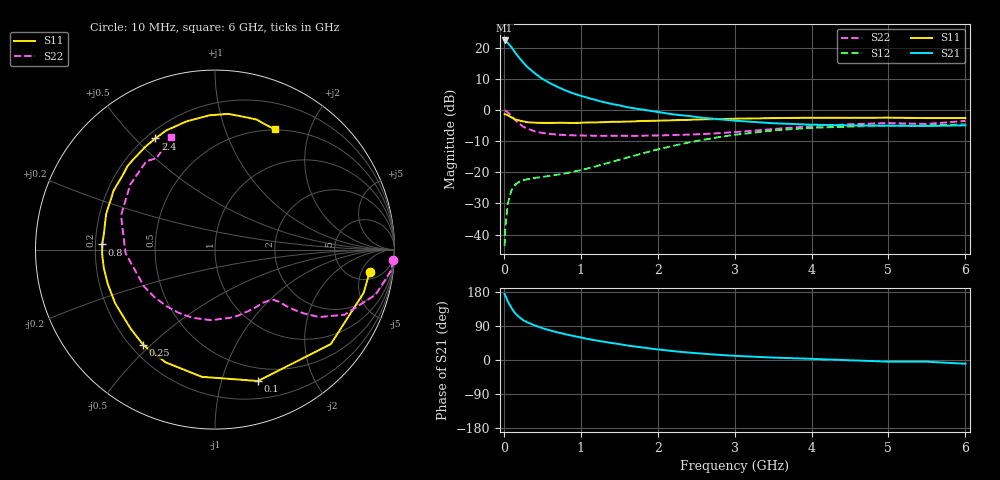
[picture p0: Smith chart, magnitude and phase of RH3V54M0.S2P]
! SIEMENS Small Signal Semiconductors
! BFR106
! Si NPN RF Bipolar Junction Transistor in SOT23
! VCE = 3.5 V  IC = 4 mA
! Common Emitter S-Parameters:  August  1996
# GHz  S  MA  R  50
!  f  S11  S21  S12  S22
! GHz  MAG  ANG  MAG  ANG  MAG  ANG  MAG  ANG
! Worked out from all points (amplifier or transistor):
!   36 points, 10 MHz to 6 GHz, reference 50 ohm
!   highest |S21| = 22.5 dB at 10 MHz (marker M1)
!   |S21| within 3 dB of that: start of sweep to 122.3 MHz
!   unconditionally stable (mu >= 1): 673.4 MHz to 1.999 GHz; 4.374 GHz to end of sweep
!   at 250 MHz: K = 0.44, MSG = 19.0 dB, |S12| = -22.5 dB
!   at 1.4 GHz: K = 1.16, MAG = 6.9 dB, |S12| = -16.6 dB
!   at 6 GHz: K = 1.02, MAG = -1.1 dB, |S12| = -4.5 dB
!   S11 on the Smith chart (normalised r, x): 10 MHz: 6.92, -7.17; 100 MHz: 0.36, -1.31; 250 MHz: 0.25, -0.47; 800 MHz: 0.23, +0.02; 2.4 GHz: 0.23, +0.57; 6 GHz: 0.49, +1.50
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0.01  0.8703 -8.3  13.32 174.2  0.0065 87.7  0.9946 -3.5
0.02  0.8628 -16.2  13.11 169.9  0.0132 80.4  0.9878 -6.8
0.05  0.8328 -39.2  12.18 155.2  0.0309 70.0  0.9295 -15.7
0.1  0.7703 -71.9  10.35 136.9  0.0522 55.6  0.8077 -26.7
0.15  0.7125 -96.0  8.408 122.5  0.064 45.4  0.6919 -32.9
0.2  0.6856 -113.8  7.021 113.2  0.0707 40.4  0.6122 -35.6
0.25  0.6647 -127.0  5.913 105.4  0.0749 36.9  0.5486 -37.4
0.3  0.644 -136.9  5.074 100.0  0.0773 35.9  0.5104 -38.3
0.4  0.6316 -151.7  3.962 91.4  0.0815 34.9  0.4598 -39.2
0.5  0.6274 -161.9  3.217 84.1  0.0846 36.3  0.4316 -40.5
0.6  0.6278 -170.4  2.733 78.1  0.0883 38.9  0.4164 -42.6
0.8  0.6292 177.4  2.093 68.0  0.0966 44.9  0.3988 -47.9
1.1  0.6377 162.1  1.577 55.3  0.1168 53.9  0.3913 -58.2
1.3  0.6438 154.1  1.355 48.1  0.1363 58.5  0.3878 -66.0
1.6  0.6569 143.5  1.127 38.4  0.1731 62.0  0.3887 -79.0
2.2  0.6922 124.0  0.862 23.5  0.268 59.9  0.4001 -108.6
2.4  0.7028 118.2  0.811 19.6  0.3027 57.3  0.4064 -120.2
3.5  0.7488 92.4  0.619 6.4  0.4743 36.4  0.4986 -177.7
4.5  0.7569 78.1  0.571 -0.7  0.5475 16.5  0.5957 142.3
5  0.7608 72.4  0.566 -4.4  0.5626 8.5  0.6236 127.8
5.5  0.7498 67.0  0.559 -4.5  0.5701 4.6  0.6043 122.6
6  0.7493 63.6  0.573 -9.9  0.5958 -3.3  0.6749 111.2
